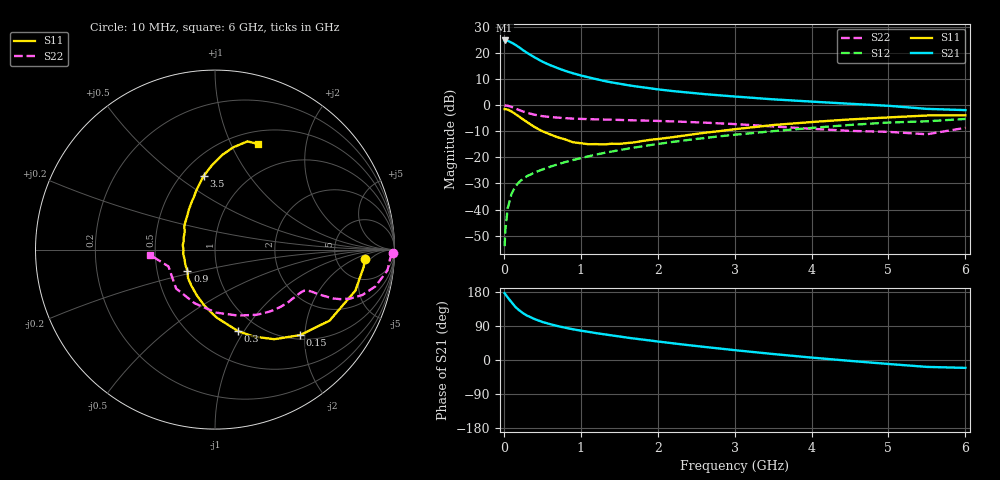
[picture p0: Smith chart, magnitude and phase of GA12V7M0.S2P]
! Infineon Technologies  Discrete & RF Semiconductors
! BF775
! Si NPN RF Bipolar Junction Transistor in SOT23
! VCE = 12 V  IC = 7 mA
! Common Emitter S-Parameters:  May  1996
# GHz  S  MA  R  50
!  f  S11  S21  S12  S22
! GHz  MAG  ANG  MAG  ANG  MAG  ANG  MAG  ANG
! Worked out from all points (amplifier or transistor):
!   36 points, 10 MHz to 6 GHz, reference 50 ohm
!   highest |S21| = 24.7 dB at 10 MHz (marker M1)
!   |S21| within 3 dB of that: start of sweep to 216.9 MHz
!   unconditionally stable (mu >= 1): 773 MHz to 2.82 GHz
!   at 250 MHz: K = 0.55, MSG = 24.6 dB, |S12| = -28.2 dB
!   at 1.4 GHz: K = 1.09, MAG = 11.4 dB, |S12| = -17.8 dB
!   at 6 GHz: K = 0.86, MSG = 1.7 dB, |S12| = -5.3 dB
!   S11 on the Smith chart (normalised r, x): 10 MHz: 10, -3; 150 MHz: 1.09, -1.89; 300 MHz: 0.80, -0.94; 900 MHz: 0.72, -0.18; 3.5 GHz: 0.64, +0.63; 6 GHz: 0.64, +1.27
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0.01  0.8362 -3.4  17.12 176.4  0.002 86.5  0.9892 -1.2
0.02  0.8338 -6.7  17.05 173.4  0.0041 82.2  0.9777 -2.8
0.05  0.8149 -16.3  16.87 165.2  0.0106 81.4  0.9677 -6.9
0.1  0.7511 -31.8  15.59 152.4  0.02 73.0  0.9171 -12.9
0.15  0.6717 -45.2  14.12 140.1  0.0277 68.2  0.8579 -17.2
0.2  0.5987 -56.5  12.65 131.1  0.0338 65.4  0.7994 -20.0
0.25  0.5306 -66.0  11.16 123.6  0.0388 62.6  0.7498 -21.6
0.3  0.4722 -74.2  9.975 117.3  0.0434 61.7  0.7106 -22.5
0.4  0.3785 -88.7  8.135 108.1  0.0512 60.8  0.6509 -23.1
0.5  0.3159 -101.1  6.741 100.4  0.0584 61.1  0.6119 -23.4
0.6  0.2746 -111.6  5.788 94.7  0.0659 61.5  0.5894 -23.5
0.7  0.2414 -122.7  5.067 89.6  0.0732 62.2  0.5732 -23.7
0.9  0.1936 -142.4  4.03 81.0  0.0888 63.1  0.5491 -24.6
1.1  0.1778 -163.0  3.379 74.3  0.1044 63.3  0.5362 -26.3
1.3  0.1756 179.9  2.89 68.0  0.1209 63.1  0.5266 -28.3
1.6  0.187 159.1  2.407 59.2  0.1452 61.9  0.5127 -31.9
2.2  0.243 129.7  1.843 44.0  0.1972 58.7  0.4854 -41.0
2.8  0.316 111.8  1.531 30.4  0.2514 53.9  0.4454 -52.6
3.5  0.4138 98.9  1.283 15.8  0.316 46.8  0.3889 -70.9
4.5  0.53 85.5  1.055 -2.3  0.4153 35.2  0.3199 -110.7
5.5  0.6295 73.3  0.843 -18.2  0.4879 20.0  0.2757 -160.2
6  0.6353 68.1  0.798 -20.8  0.5408 15.8  0.366 -175.6
